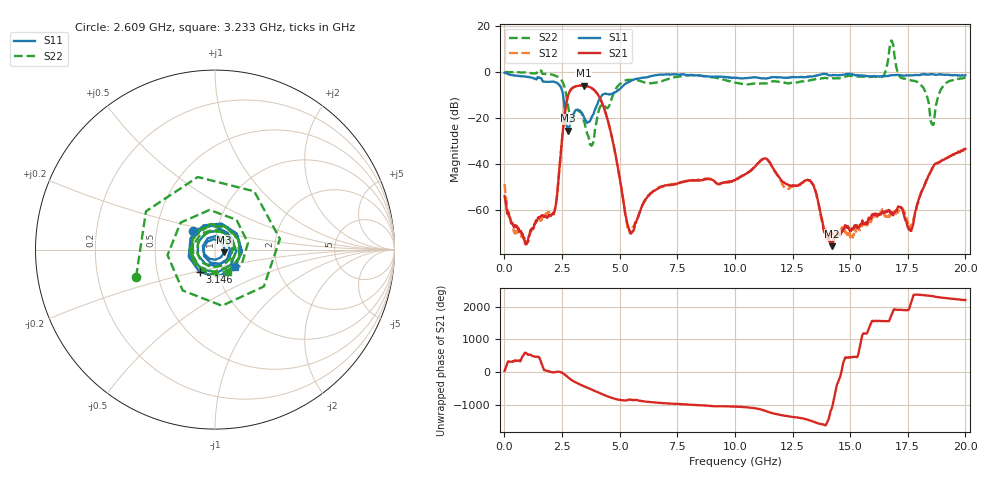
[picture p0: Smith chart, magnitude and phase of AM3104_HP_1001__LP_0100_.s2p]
!Created with skrf (http://scikit-rf.org).
# Hz S RI R 50.0
!freq ReS11 ImS11 ReS21 ImS21 ReS12 ImS12 ReS22 ImS22
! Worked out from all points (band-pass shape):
!   1601 points, 10 MHz to 20 GHz, reference 50 ohm
!   highest |S21| = -5.91 dB at 3.433 GHz (marker M1); lowest = -75.6 dB at 14.22 GHz (marker M2)
!   |S21| within 3 dB of the highest: 2.812 GHz to 3.992 GHz (1.18 GHz wide, 34.7 % of centre)
!   lowest |S11| = -25.5 dB at 2.771 GHz (marker M3), VSWR 1.11, Z = 55.3 - j1.7 ohm
!   |S11| at or under -10 dB: 2.547 GHz to 4.247 GHz (1.7 GHz wide, 50.1 % of centre)
!   |S22| runs from -32.1 to 13.7 dB; largest |S21 - S12| = 0.025
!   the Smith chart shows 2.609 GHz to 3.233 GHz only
!   S11 on the Smith chart (normalised r, x): 2.609 GHz: 0.77, +0.17; 3.146 GHz: 0.82, -0.21; 3.233 GHz: 1.22, -0.24
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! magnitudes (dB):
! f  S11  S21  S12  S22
! 10 MHz  -0.4  -54.0  -48.8  0.0
! 959.5 MHz  -2.1  -74.5  -73.7  -0.2
! 2.109 GHz  -4.2  -61.5  -61.8  -1.2
! 2.609 GHz  -15.8  -19.1  -19.1  -6.7
! 2.771 GHz  -25.5  -10.0  -10.0  -15.3
! 3.146 GHz  -16.4  -6.1  -6.1  -17.0
! 3.233 GHz  -16.7  -6.0  -6.0  -17.0
! 3.346 GHz  -17.6  -5.9  -6.0  -17.8
! 3.433 GHz  -19.3  -5.9  -5.9  -20.8
! 3.783 GHz  -19.7  -7.0  -7.0  -32.1
! 4.383 GHz  -9.4  -17.6  -17.6  -15.3
! 5.432 GHz  -4.2  -68.8  -69.3  -3.4
! 6.682 GHz  -1.2  -50.5  -50.2  -4.5
! 10.01 GHz  -2.6  -47.1  -46.9  -4.7
! 11.32 GHz  -2.9  -37.6  -37.8  -5.0
! 13.34 GHz  -2.0  -48.2  -48.2  -3.5
! 14.22 GHz  -1.5  -75.6  -70.0  -2.8
! 16.68 GHz  -1.6  -60.3  -64.1  7.2
! 17.64 GHz  -1.4  -68.9  -67.6  -3.6
! 18.56 GHz  -0.9  -41.7  -42.0  -22.7
! 19.03 GHz  -1.2  -38.2  -38.0  -6.3
! 20 GHz  -1.4  -33.5  -33.1  -2.5
